PROGRAM MAIN
VAR
	////////////////////////模式//////////////////////////////////////////
	mode_state:INT;
END_VAR

IF mode_state=0 THEN
	Mannual();
END_IF
IF mode_state=1 THEN
	Auto();
END_IF

END_PROGRAM
